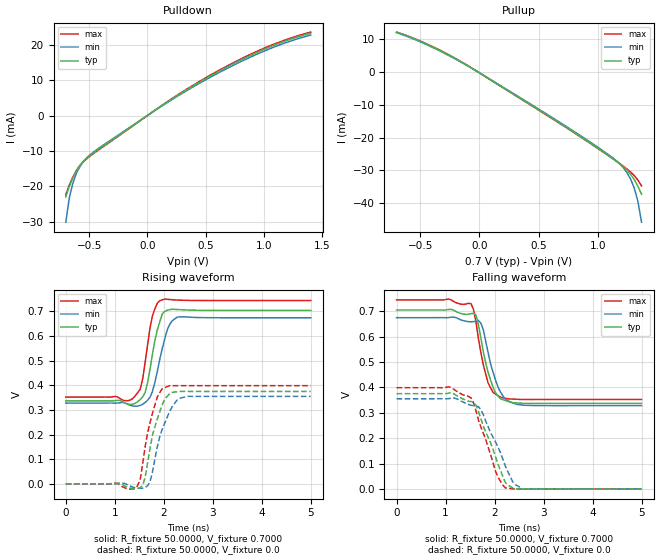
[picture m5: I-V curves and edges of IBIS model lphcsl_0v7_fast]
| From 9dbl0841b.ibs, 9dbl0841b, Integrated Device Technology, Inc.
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|   Model lphcsl_0v7_fast
[Model]  lphcsl_0v7_fast
Model_type Output
Polarity   Non-Inverting
Vmeas =  0.4000V
Cref =   2.0000pF
Rref =   0.0
Vref =   0.4000V
C_comp   1.1000pF   1.0000pF   1.2000pF
[Temperature Range]   27.0000   70.0000   0.0
[Voltage Range]   0.7000V   0.6700V   0.7400V
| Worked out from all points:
|   slope of the pulldown table from 0 to 0.105 V, typ, clamps not added: 44.3 ohm
|   slope of the pullup table from 0 to 0.105 V, typ, clamps not added: 44.4 ohm
|   rising waveform, R_fixture 50.0000, V_fixture 0.7000: 20-80 % time 208ps typ, 244ps min, 180ps max; typ from 0.337 V to 0.704 V
|   rising waveform, R_fixture 50.0000, V_fixture 0.0: 20-80 % time 269ps typ, 308ps min, 248ps max; typ from 0 V to 0.375 V
|   falling waveform, R_fixture 50.0000, V_fixture 0.7000: 20-80 % time 266ps typ, 286ps min, 237ps max; typ from 0.704 V to 0.337 V
|   falling waveform, R_fixture 50.0000, V_fixture 0.0: 20-80 % time 437ps typ, 476ps min, 402ps max; typ from 0.375 V to 0 V
[Pulldown]
|Voltage   I(typ)   I(min)   I(max)
-700mV    -23mA      -30.13mA   -22.37mA
-670mV    -20.06mA   -23.34mA   -19.68mA
-640mV    -17.66mA   -19.18mA   -17.42mA
-610mV    -15.72mA   -16.44mA   -15.59mA
-550mV    -12.99mA   -13.03mA   -13.08mA
-460mV    -10.5mA    -10.25mA   -10.7mA
170mV     3.791mA    3.653mA    3.891mA
530mV     10.98mA    10.63mA    11.23mA
800mV     15.65mA    15.2mA     15.96mA
1.01V     18.83mA    18.32mA    19.15mA
1.22V     21.47mA    20.95mA    21.77mA
1.4V      23.24mA    22.71mA    23.56mA
[Pullup]
|Voltage   I(typ)   I(min)   I(max)
-700mV    12.25mA    12.08mA    12.21mA
-430mV    8.33mA     8.148mA    8.393mA
-130mV    2.65mA     2.576mA    2.694mA
650mV     -14.87mA   -14.61mA   -14.98mA
920mV     -21.21mA   -20.93mA   -21.31mA
1.13V     -26.43mA   -26.22mA   -26.47mA
1.22V     -28.93mA   -29.29mA   -28.78mA
1.25V     -29.97mA   -30.81mA   -29.61mA
1.28V     -31.24mA   -32.79mA   -30.52mA
1.31V     -32.85mA   -35.5mA    -31.6mA
1.34V     -34.83mA   -39.47mA   -32.96mA
1.37V     -37.24mA   -45.78mA   -34.69mA
[Ramp]
| variable   typ   min   max
dV/dt_r  0.2250/0.2692n   0.2130/0.3076n   0.2391/0.2485n
dV/dt_f  0.2205/0.2662n   0.2077/0.2862n   0.2353/0.2374n
R_load = 50.0000
[Rising Waveform]
R_fixture= 50.0000
V_fixture= 0.7000
V_fixture_min= 0.6700
V_fixture_max= 0.7400
|time   V(typ)   V(min)   V(max)
0s        336.9mV    328mV      352.2mV
1.26ns    324.1mV    323.6mV    337.5mV
1.41ns    326.1mV    315.3mV    355.3mV
1.52ns    341.9mV    318.1mV    384.8mV
1.62ns    370.6mV    330.2mV    493.6mV
1.77ns    527.2mV    375.4mV    681.8mV
1.92ns    658.4mV    506.5mV    743.7mV
2.07ns    704.7mV    625mV      749.5mV
2.27ns    707.9mV    676.3mV    746.4mV
5ns       704.4mV    674.2mV    744.4mV
[Rising Waveform]
R_fixture= 50.0000
V_fixture= 0.0
V_fixture_min= 0.0
V_fixture_max= 0.0
|time   V(typ)   V(min)   V(max)
0s        629.4nV    0V         772.1nV
1.46ns    -19.23mV   -18.03mV   -9.86mV
1.52ns    -15.35mV   -18.82mV   17.9mV
1.57ns    -6.433mV   -17.91mV   81.61mV
1.72ns    143.9mV    9.296mV    248.7mV
1.87ns    263.7mV    152mV      353mV
2.12ns    365.9mV    293.7mV    398.5mV
2.27ns    373.8mV    339.7mV    398.4mV
2.47ns    375.1mV    354.9mV    398.5mV
5ns       375mV      355mV      398.5mV
[Falling Waveform]
R_fixture= 50.0000
V_fixture= 0.7000
V_fixture_min= 0.6700
V_fixture_max= 0.7400
|time   V(typ)   V(min)   V(max)
0s        704.4mV    674.2mV    744.4mV
1.52ns    690mV      658mV      729.6mV
1.62ns    684.9mV    660.9mV    658.9mV
1.72ns    596mV      652.8mV    537.5mV
1.87ns    458.1mV    536mV      416.4mV
2.02ns    378.9mV    428.2mV    373.8mV
2.12ns    355.2mV    381.6mV    361.2mV
2.22ns    348.1mV    352.3mV    356.8mV
2.58ns    337.3mV    329.9mV    352.2mV
5ns       336.9mV    328mV      352.2mV
[Falling Waveform]
R_fixture= 50.0000
V_fixture= 0.0
V_fixture_min= 0.0
V_fixture_max= 0.0
|time   V(typ)   V(min)   V(max)
0s        375mV      355mV      398.5mV
1.06ns    377.2mV    355.3mV    402.1mV
1.52ns    344.1mV    329.6mV    358.7mV
1.62ns    330.5mV    325.8mV    308.3mV
1.72ns    276.9mV    312.1mV    244.3mV
2.02ns    126.3mV    184.8mV    69.7mV
2.22ns    25.58mV    90.69mV    4.236mV
2.37ns    4.05mV     28.51mV    544.2uV
2.58ns    94.9uV     -896.6uV   -280.6uV
5ns       737.4nV    0V         921nV
